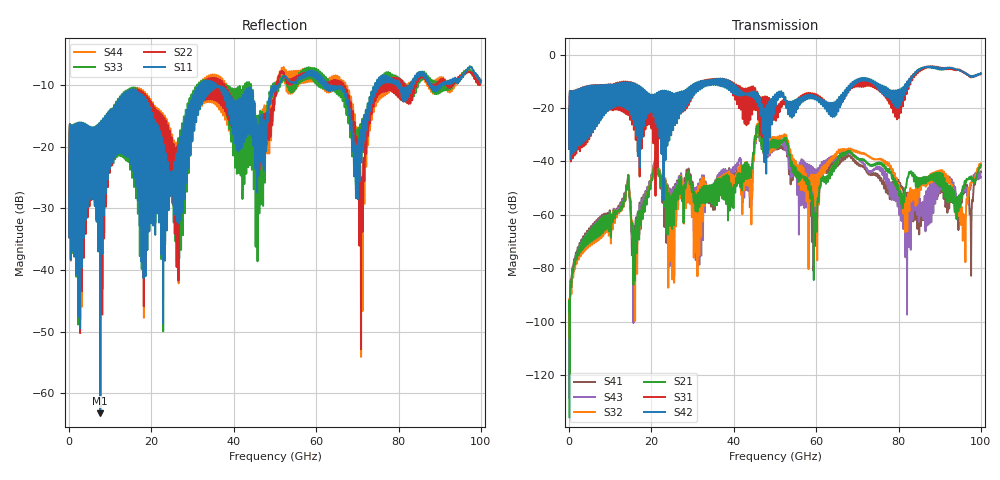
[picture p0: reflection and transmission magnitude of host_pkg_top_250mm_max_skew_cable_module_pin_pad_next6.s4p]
# Hz S RI R 50
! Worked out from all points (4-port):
!   10000 points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, 10 MHz to 100 GHz, reference 50 ohm
!   strongest paths, dB at 10 MHz, 25.01 GHz, 50.01 GHz, 75.01 GHz, 100 GHz:
!     S42: -35.3, -14.4, -15.0, -11.9, -7.0
!     S31: -35.3, -17.4, -19.3, -12.5, -7.1
!     S21: -96.5, -64.0, -34.7, -40.4, -41.4
!     S32: -96.1, -62.5, -35.0, -39.1, -40.8
!     S43: -96.4, -56.1, -35.1, -42.4, -45.9
!     S41: -96.9, -58.8, -35.1, -45.9, -44.0
!   lowest |S11| = -63.2 dB at 7.58 GHz (marker M1), VSWR 1.00, Z = 49.9 - j0.00261 ohm
!   |S11| at or under -10 dB: start of sweep to 31.92 GHz; 35.74 GHz to 50.81 GHz (15.08 GHz wide, 34.8 % of centre); 62.81 GHz to 74.31 GHz (11.5 GHz wide, 16.8 % of centre)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
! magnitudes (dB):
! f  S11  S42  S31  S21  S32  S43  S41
! 10 MHz  -34.7  -35.3  -35.3  -96.5  -96.1  -96.4  -96.9
! 7.58 GHz  -63.2  -22.4  -24.1  -61.6  -62.4  -61.4  -60.6
! 46.07 GHz  -23.3  -18.8  -16.3  -26.3  -24.8  -26.6  -28.3
! 59.79 GHz  -8.9  -16.8  -16.0  -66.2  -55.6  -60.8  -62.9
! 67.69 GHz  -12.6  -14.1  -13.6  -36.1  -35.7  -37.1  -37.7
! 82.08 GHz  -12.3  -10.2  -11.6  -46.6  -62.2  -85.3  -56.5
! 100 GHz  -9.4  -7.0  -7.1  -41.4  -40.8  -45.9  -44.0
